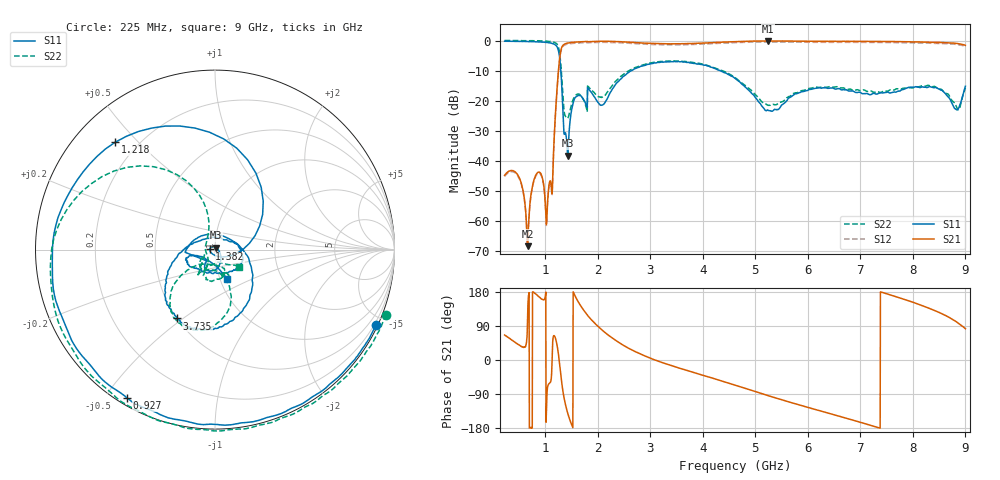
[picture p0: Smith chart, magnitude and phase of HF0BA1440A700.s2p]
!Agilent Technologies,E8358A,US41080443,A.07.50.56
!Agilent E8358A: A.07.50.56
!Date: Friday, July 08, 2016 13:14:07
!Correction: S11(Full 2 Port(1,2))
!S21(Full 2 Port(1,2))
!S12(Full 2 Port(1,2))
!S22(Full 2 Port(1,2))
!S2P File: Measurements: S11, S21, S12, S22:
# Hz S  dB  R 50
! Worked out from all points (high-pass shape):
!   1601 points, 225 MHz to 9 GHz, reference 50 ohm
!   highest |S21| = 0.04 dB at 5.238 GHz (marker M1); lowest = -68.4 dB at 663.8 MHz (marker M2)
!   |S21| within 3 dB of the highest: 1.299 GHz to end of sweep
!   lowest |S11| = -38.3 dB at 1.426 GHz (marker M3), VSWR 1.02, Z = 50.7 + j1.01 ohm
!   |S11| at or under -10 dB: 1.296 GHz to 2.628 GHz (1.332 GHz wide, 67.9 % of centre); 4.341 GHz to end of sweep
!   |S22| runs from -25.8 to 0.2 dB; largest |S21 - S12| = 0.041
!   S11 on the Smith chart (normalised r, x): 225 MHz: 0.09, -4.50; 927 MHz: 0.03, -0.57; 1.218 GHz: 0.12, +0.43; 1.382 GHz: 0.94, +0.00; 3.735 GHz: 0.50, -0.48; 9 GHz: 1.08, -0.36
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2.25e8  -0.07 -25.1  -44.78 66.1  -45.17 66.2  0.18 -20.8
4.992188e8  -0.15 -56.8  -45.48 39.7  -45.79 39.8  0.12 -47.2
6.6375e8  -0.16 -78.2  -68.43 119.6  -67.85 116.8  0.12 -65.2
7.844062e8  -0.20 -95.6  -46.28 178.1  -46.64 178.2  0.11 -80.0
9.27e8  -0.35 -120.8  -44.68 160.7  -45.02 161.2  0.03 -101.1
1.053141e9  -0.55 -150.6  -50.96 -66.3  -51.40 -66.2  -0.11 -125.3
1.135406e9  -0.85 -178.6  -48.83 30.9  -49.09 30.5  -0.28 -147.1
1.217672e9  -1.76 132.9  -17.43 43.5  -17.77 43.8  -0.91 176.5
1.294453e9  -9.62 36.5  -3.33 -38.3  -3.67 -38.1  -7.66 112.5
1.382203e9  -30.59 176.0  -0.90 -116.5  -1.25 -116.4  -25.07 165.0
1.426078e9  -38.27 54.9  -0.67 -140.2  -1.01 -139.9  -25.75 -153.9
1.54125e9  -20.01 -79.7  -0.40 176.5  -0.75 176.7  -19.06 -115.6
1.689328e9  -18.52 -118.6  -0.25 139.7  -0.59 139.9  -18.40 -135.1
2.352938e9  -14.12 -15.9  -0.19 50.6  -0.53 50.7  -13.19 -68.6
3.153656e9  -7.15 -89.5  -0.86 -3.3  -1.21 -3.1  -6.89 -98.0
3.735e9  -7.17 -118.9  -0.83 -29.2  -1.18 -29.2  -6.99 -119.1
4.6125e9  -12.47 -164.5  -0.22 -66.1  -0.55 -66.0  -12.19 -142.2
5.237719e9  -23.07 101.5  0.04 -93.7  -0.31 -93.7  -21.42 -105.0
6.076828e9  -16.06 -14.1  -0.08 -127.9  -0.43 -128.0  -15.74 -62.4
7.541156e9  -17.20 -123.1  -0.17 173.0  -0.49 172.9  -16.57 -74.7
8.829984e9  -22.90 -127.9  -0.79 100.7  -1.13 100.6  -21.93 -92.7
9e9  -15.10 -67.9  -1.45 82.5  -1.78 82.2  -15.68 -36.1
